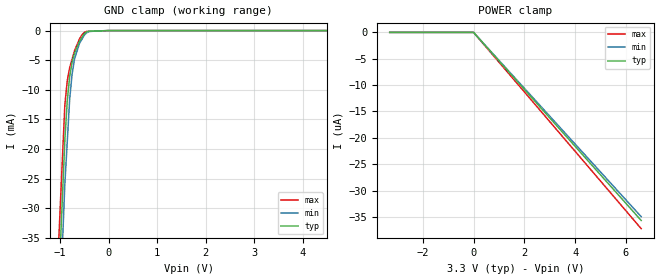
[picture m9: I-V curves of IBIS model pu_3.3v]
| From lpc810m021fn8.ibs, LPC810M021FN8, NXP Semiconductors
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[Model] pu_3.3v
Model_type Input
Vinl = 990.000mV
Vinh = 2.31000V
C_comp 909.000fF 904.000fF 914.000fF
| variable typ   min   max
[Voltage Range] 3.30000V 3.00000V 3.60000V
[POWER Clamp Reference] 3.30000V 3.00000V 3.60000V
[GND Clamp Reference] 0.00000V 0.00000V 0.00000V
[Temperature Range]   25   85   -40
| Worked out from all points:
|   GND clamp passes 1 mA (typ) near -0.54 V on its own axis
[GND Clamp]
-3.3V     -481.7mA   -520.5mA   -449mA
-900mV    -18.53mA   -25.95mA   -12.56mA
-850mV    -11.85mA   -18.75mA   -8.473mA
-800mV    -7.74mA    -11.54mA   -6.254mA
-750mV    -5.325mA   -7.326mA   -4.829mA
-700mV    -3.812mA   -4.773mA   -3.403mA
-600mV    -1.827mA   -2.206mA   -1.457mA
-550mV    -1.183mA   -1.492mA   -748.6uA
-450mV    -225.2uA   -371.1uA   -135.9uA
-400mV    -100.7uA   -153.2uA   -124uA
0V        0A         0A         0A
6.6V      0A         0A         0A
[POWER Clamp]
-3.3V     0A         0A         0A
0V        0A         0A         0A
6.6V      -35.67uA   -34.94uA   -37.22uA
